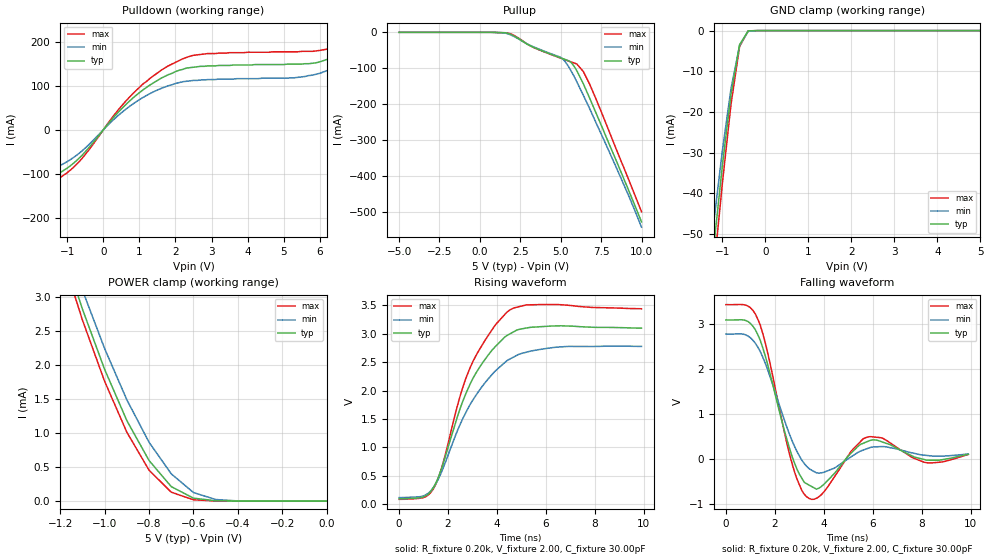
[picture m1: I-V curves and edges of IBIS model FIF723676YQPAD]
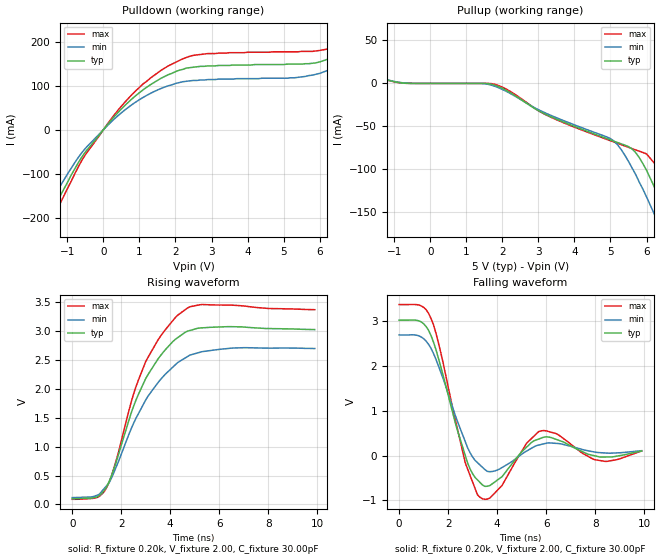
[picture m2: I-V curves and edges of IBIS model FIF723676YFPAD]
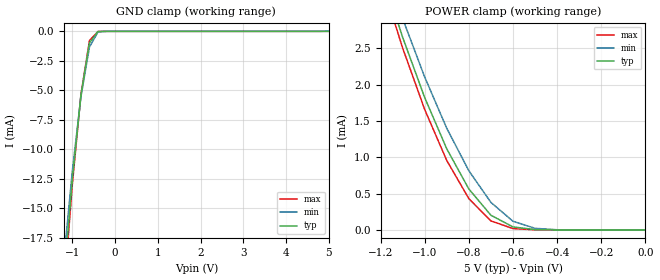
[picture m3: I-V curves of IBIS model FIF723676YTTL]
| IBIS file f723676.ibs created by s2ibis2 version 1.1
| North Carolina State University Electronics Research Laboratory  1995
[IBIS ver]   2.1
[File name]   f723676.ibs
[File Rev]   1.0
[Date]   05/05/99
[Source]   Integrated Device Technology, Inc.
[Notes]   1. Temperatures: typ=25C, min=70C, max=0C 2. Cemos9_5v
   process. 3. Ramp rates based on 50 ohm load.
[Copyright]   Copyright 1999, Integrated Device Technology, Inc.
|   Component idt723676y
[Component]   idt723676y
[Manufacturer]   Integrated Device Technology
[Package]
| variable   typ   min   max
R_pkg   0.75   0.60   0.90
L_pkg   8.10nH   8.30nH   9.90nH
C_pkg   0.53pF   0.46pF   0.60pF
[Pin]  signal_name   model_name   R_pin   L_pin   C_pin
1   WRLA   FIF723676YTTL
2   ENA   FIF723676YTTL
3   CLKA   FIF723676YTTL
4   GND   GND
5   A35   FIF723676YQPAD
6   A34   FIF723676YQPAD
7   A33   FIF723676YQPAD
8   A32   FIF723676YQPAD
9   VCC   POWER
10   A31   FIF723676YQPAD
11   A30   FIF723676YQPAD
12   GND   GND
13   A29   FIF723676YQPAD
14   A28   FIF723676YQPAD
15   A27   FIF723676YQPAD
16   A26   FIF723676YQPAD
17   A25   FIF723676YQPAD
18   A24   FIF723676YQPAD
19   A23   FIF723676YQPAD
20   BEFWFTL   FIF723676YTTL
21   GND   GND
22   A22   FIF723676YQPAD
23   VCC   POWER
24   A21   FIF723676YQPAD
25   A20   FIF723676YQPAD
26   A19   FIF723676YQPAD
27   A18   FIF723676YQPAD
28   GND   GND
29   A17   FIF723676YQPAD
30   A16   FIF723676YQPAD
31   A15   FIF723676YQPAD
32   A14   FIF723676YQPAD
33   A13   FIF723676YQPAD
34   VCC   POWER
35   A12   FIF723676YQPAD
36   GND   GND
37   A11   FIF723676YQPAD
38   A10   FIF723676YQPAD
39   A9   FIF723676YQPAD
40   A8   FIF723676YQPAD
41   A7   FIF723676YQPAD
42   A6   FIF723676YQPAD
43   GND   GND
44   A5   FIF723676YQPAD
45   A4   FIF723676YQPAD
46   A3   FIF723676YQPAD
47   FS2   FIF723676YTTL
48   VCC   POWER
49   A2   FIF723676YQPAD
50   A1   FIF723676YQPAD
51   A0   FIF723676YQPAD
52   GND   GND
53   B0   FIF723676YQPAD
54   B1   FIF723676YQPAD
55   B2   FIF723676YQPAD
56   B3   FIF723676YQPAD
57   B4   FIF723676YQPAD
58   B5   FIF723676YQPAD
59   GND   GND
60   B6   FIF723676YQPAD
61   VCC   POWER
62   B7   FIF723676YQPAD
63   B8   FIF723676YQPAD
64   B9   FIF723676YQPAD
65   B10   FIF723676YQPAD
66   B11   FIF723676YQPAD
67   GND   GND
68   B12   FIF723676YQPAD
69   B13   FIF723676YQPAD
70   B14   FIF723676YQPAD
71   B15   FIF723676YQPAD
72   VCC   POWER
73   SIZEC   FIF723676YTTL
74   B16   FIF723676YQPAD
75   B17   FIF723676YQPAD
76   GND   GND
77   C0   FIF723676YQPAD
78   C1   FIF723676YQPAD
79   C2   FIF723676YQPAD
80   C3   FIF723676YQPAD
81   C4   FIF723676YQPAD
82   C5   FIF723676YQPAD
83   GND   GND
84   SIZEB   FIF723676YTTL
85   C6   FIF723676YQPAD
86   C7   FIF723676YQPAD
87   VCC   POWER
88   C8   FIF723676YQPAD
89   C9   FIF723676YQPAD
90   C10   FIF723676YQPAD
91   C11   FIF723676YQPAD
92   C12   FIF723676YQPAD
93   C13   FIF723676YQPAD
94   MBC   FIF723676YTTL
95   RTM   FIF723676YTTL
96   C14   FIF723676YQPAD
97   C15   FIF723676YQPAD
98   C16   FIF723676YQPAD
99   C17   FIF723676YQPAD
100   LOOPL   FIF723676YTTL
101   PRS2L   FIF723676YTTL
102   CLKB   FIF723676YTTL
103   ENB   FIF723676YTTL
104   WLRB   FIF723676YTTL
105   CSBL   FIF723676YTTL
106   GND   GND
107   IRFFLC   FIF723676YFPAD
108   OREFLB   FIF723676YFPAD
109   AFCL   FIF723676YFPAD
110   AEBL   FIF723676YFPAD
111   VCC   POWER
112   MBF1L   FIF723676YFPAD
113   MBB   FIF723676YTTL
114   MRS2L   FIF723676YTTL
115   FS1SENL   FIF723676YTTL
116   GND   GND
117   CLKC   FIF723676YTTL
118   FS0SD   FIF723676YTTL
119   MRS1L   FIF723676YTTL
120   MBA   FIF723676YTTL
121   MBF2L   FIF723676YFPAD
122   AEAL   FIF723676YFPAD
123   AFAL   FIF723676YFPAD
124   VCC   POWER
125   PRS1L   FIF723676YTTL
126   OREFLA   FIF723676YFPAD
127   IRFFLA   FIF723676YFPAD
128   CSAL   FIF723676YTTL
| Models and submodels in the file (3): FIF723676YQPAD (I/O), FIF723676YFPAD (Output), FIF723676YTTL (Input)
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| FIN  FIN   dummy_model
| QIN  QIN   dummy_model
| QOEL QOEL   dummy_model
|   Model FIF723676YQPAD
[Model]   FIF723676YQPAD
Model_type   I/O
Polarity   Non-Inverting
Enable   Active-Low
Vinl =  0.000V
Vinh =  3.000V
Vmeas =  1.500V
C_comp   3.00pF   NA   NA
[Temperature Range]   25.00   70.00   0.000
[Voltage Range]   5.00V   4.50V   5.50V
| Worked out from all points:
|   slope of the pulldown table from 0 to 0.75 V, typ, clamps not added: 11.2 ohm
|   slope of the pullup table from 0 to 0.75 V, typ, clamps not added: 24.4 kohm
|   GND clamp passes 1 mA (typ) near -0.45 V on its own axis
|   POWER clamp passes 1 mA (typ) near -0.87 V on its own axis
|   rising waveform, R_fixture 0.20k, V_fixture 2.00, C_fixture 30.00pF: 20-80 % time 1.64ns typ, 1.91ns min, 1.53ns max; typ from 0.099 V to 3.1 V
|   falling waveform, R_fixture 0.20k, V_fixture 2.00, C_fixture 30.00pF: 20-80 % time 861ps typ, 1.01ns min, 804ps max; typ from 3.1 V to 0.103 V
[Pulldown]
| voltage   I(typ)   I(min)   I(max)
-5V       -212mA     -180mA     -238mA
-2.6V     -150mA     -127mA     -168mA
-1.4V     -108mA     -90.18mA   -120mA
-600mV    -58.74mA   -48.6mA    -65.88mA
900mV     77.62mA    63.02mA    88.53mA
2.2V      137mA      109mA      161mA
5.8V      151mA      124mA      178mA
6.4V      165mA      140mA      186mA
6.8V      189mA      163mA      206mA
7.2V      235mA      207mA      249mA
7.6V      322mA      286mA      332mA
10V       3.398A     2.916A     3.573A
[Pullup]
| voltage   I(typ)   I(min)   I(max)
-5V       0A         0A         0A
700mV     -2.902uA   -34.47uA   -378nA
1.7V      -2.465mA   -3.753mA   -1.627mA
2.2V      -12.35mA   -13.59mA   -10.75mA
3.3V      -41.26mA   -40.02mA   -41.62mA
5.1V      -72.73mA   -73.03mA   -73.46mA
5.7V      -86.77mA   -112mA     -83.28mA
6V        -107mA     -138mA     -88.21mA
6.4V      -143mA     -175mA     -109mA
7.2V      -226mA     -253mA     -187mA
9.2V      -439mA     -454mA     -409mA
10V       -527mA     -542mA     -499mA
[GND_clamp]
| voltage   I(typ)   I(min)   I(max)
-5V       -521mA     -479mA     -549mA
-1.4V     -74.67mA   -66.42mA   -82.01mA
-1.2V     -53.14mA   -47.16mA   -59.1mA
-1V       -33.18mA   -29.54mA   -37.54mA
-800mV    -15.68mA   -14.32mA   -18.21mA
-600mV    -3.449mA   -3.672mA   -3.919mA
-400mV    -78.08uA   -158uA     -61.68uA
-200mV    -109nA     -686nA     -39.2nA
5V        50.13nA    23.69uA    50.08nA
[POWER_clamp]
| voltage   I(typ)   I(min)   I(max)
-5V       61.91mA    58.94mA    63.83mA
-1.2V     3.823mA    4.054mA    3.693mA
-1.1V     2.823mA    3.102mA    2.663mA
-1V       1.936mA    2.242mA    1.761mA
-900mV    1.184mA    1.489mA    1.013mA
-800mV    597uA      865uA      455uA
-700mV    213uA      401uA      131uA
-600mV    43.85uA    126uA      19.94uA
-500mV    5.315uA    23.69uA    1.903uA
-400mV    453nA      2.906uA    155nA
0V        50.13nA    46.03nA    55.09nA
[Ramp]
| variable   typ   min   max
dV/dt_r   1.12/0.84n   0.95/1.02n   1.28/0.75n
dV/dt_f   2.43/0.80n   2.09/1.03n   2.74/0.70n
R_load = 50.00
[Rising Waveform]
R_fixture = 0.20k
V_fixture = 2.00
C_fixture = 30.00pF
R_dut = 0.75
L_dut = 8.10nH
C_dut = 0.53pF
| time   V(typ)   V(min)   V(max)
0s        99.01mV    119mV      88.78mV
1ns       132mV      149mV      120mV
1.4ns     294mV      296mV      272mV
1.7ns     589mV      534mV      585mV
2.5ns     1.693V     1.412V     1.913V
2.9ns     2.114V     1.754V     2.399V
3.7ns     2.657V     2.234V     3.006V
4.5ns     2.989V     2.548V     3.409V
6.4ns     3.135V     2.76V      3.511V
9.9ns     3.096V     2.775V     3.436V
[Falling Waveform]
R_fixture = 0.20k
V_fixture = 2.00
C_fixture = 30.00pF
R_dut = 0.75
L_dut = 8.10nH
C_dut = 0.53pF
| time   V(typ)   V(min)   V(max)
0s        3.098V     2.784V     3.44V
900ps     3.064V     2.74V      3.408V
1.3ns     2.774V     2.496V     3.117V
1.7ns     2.117V     1.997V     2.378V
2.7ns     59mV       407mV      -98.99mV
3.4ns     -586mV     -218mV     -884mV
3.9ns     -616mV     -312mV     -797mV
5.8ns     391mV      235mV      490mV
8.1ns     -14.31mV   82.42mV    -76.01mV
9.9ns     103mV      109mV      98.9mV
|   Model FIF723676YFPAD
[Model]   FIF723676YFPAD
Model_type   Output
Vmeas =  1.500V
C_comp   3.00pF   NA   NA
[Temperature Range]   25.00   70.00   0.000
[Voltage Range]   5.00V   4.50V   5.50V
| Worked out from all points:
|   slope of the pulldown table from 0 to 0.75 V, typ, clamps not added: 11.2 ohm
|   rising waveform, R_fixture 0.20k, V_fixture 2.00, C_fixture 30.00pF: 20-80 % time 1.63ns typ, 1.87ns min, 1.54ns max; typ from 0.099 V to 3.03 V
|   falling waveform, R_fixture 0.20k, V_fixture 2.00, C_fixture 30.00pF: 20-80 % time 856ps typ, 994ps min, 801ps max; typ from 3.03 V to 0.107 V
[Pulldown]
| voltage   I(typ)   I(min)   I(max)
-5V       -725mA     -652mA     -779mA
-2.2V     -305mA     -267mA     -333mA
-1.8V     -243mA     -211mA     -267mA
-1.4V     -181mA     -155mA     -201mA
-700mV    -75.3mA    -63.31mA   -84.95mA
300mV     29.64mA    24.2mA     33.55mA
2.2V      137mA      109mA      161mA
5.8V      151mA      124mA      178mA
6.8V      189mA      163mA      206mA
7.2V      235mA      207mA      249mA
7.6V      322mA      286mA      332mA
10V       3.398A     2.916A     3.573A
[Pullup]
| voltage   I(typ)   I(min)   I(max)
-5V       61.91mA    58.94mA    63.83mA
-1V       1.936mA    2.242mA    1.761mA
1.8V      -2.262mA   -3.492mA   -1.177mA
3.2V      -35.97mA   -34.51mA   -36.4mA
5V        -65.77mA   -64.22mA   -66.68mA
5.3V      -70.31mA   -77.14mA   -71.29mA
5.7V      -80.57mA   -106mA     -77.38mA
6V        -101mA     -132mA     -81.97mA
6.4V      -137mA     -169mA     -102mA
6.8V      -178mA     -208mA     -139mA
7.2V      -219mA     -247mA     -181mA
10V       -520mA     -534mA     -490mA
[Ramp]
| variable   typ   min   max
dV/dt_r   1.08/0.85n   0.91/1.00n   1.23/0.75n
dV/dt_f   2.43/0.76n   2.09/0.94n   2.74/0.67n
R_load = 50.00
[Rising Waveform]
R_fixture = 0.20k
V_fixture = 2.00
C_fixture = 30.00pF
R_dut = 0.75
L_dut = 8.10nH
C_dut = 0.53pF
| time   V(typ)   V(min)   V(max)
0s        99.01mV    119mV      88.78mV
1ns       130mV      158mV      118mV
1.4ns     302mV      323mV      291mV
1.8ns     743mV      656mV      775mV
2.5ns     1.697V     1.404V     1.91V
3ns       2.182V     1.812V     2.477V
3.6ns     2.577V     2.163V     2.912V
4.3ns     2.888V     2.457V     3.277V
5.3ns     3.06V      2.647V     3.464V
9.9ns     3.029V     2.701V     3.374V
[Falling Waveform]
R_fixture = 0.20k
V_fixture = 2.00
C_fixture = 30.00pF
R_dut = 0.75
L_dut = 8.10nH
C_dut = 0.53pF
| time   V(typ)   V(min)   V(max)
0s        3.028V     2.697V     3.376V
900ps     2.989V     2.653V     3.346V
1.3ns     2.685V     2.4V       3.066V
2.7ns     5.93mV     314mV      -160mV
3.3ns     -597mV     -207mV     -928mV
4.2ns     -468mV     -264mV     -666mV
5.2ns     190mV      103mV      277mV
5.8ns     394mV      252mV      556mV
8ns       -3.386mV   80.65mV    -90.39mV
9.9ns     107mV      113mV      106mV
|   Model FIF723676YTTL
[Model]   FIF723676YTTL
Model_type   Input
Vinl =  0.000V
Vinh =  3.000V
Vmeas =  1.500V
C_comp   3.00pF   NA   NA
[Temperature Range]   25.00   70.00   0.000
[Voltage Range]   5.00V   4.50V   5.50V
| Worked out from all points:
|   GND clamp passes 1 mA (typ) near -0.60 V on its own axis
|   POWER clamp passes 1 mA (typ) near -0.88 V on its own axis
[GND_clamp]
| voltage   I(typ)   I(min)   I(max)
-5V       -230mA     -211mA     -242mA
-1.2V     -21.09mA   -19.36mA   -22.25mA
-1V       -12.49mA   -11.81mA   -12.95mA
-800mV    -5.437mA   -5.552mA   -5.361mA
-600mV    -980uA     -1.334mA   -778uA
-400mV    -16.84uA   -48.96uA   -8uA
5V        50.08nA    22.72uA    50.04nA
[POWER_clamp]
| voltage   I(typ)   I(min)   I(max)
-5V       58.05mA    55.22mA    59.87mA
-1.2V     3.594mA    3.805mA    3.475mA
-1.1V     2.656mA    2.913mA    2.508mA
-1V       1.824mA    2.107mA    1.66mA
-900mV    1.118mA    1.401mA    957uA
-800mV    565uA      816uA      432uA
-700mV    203uA      380uA      125uA
-600mV    42.07uA    120uA      19.22uA
-500mV    5.131uA    22.72uA    1.847uA
-400mV    442nA      2.801uA    153nA
0V        50.08nA    45.71nA    55.05nA
